(* Logix 5000 AddOnInstructionDefinition export AMCI_3202_AOP_Immediate_Stop; software revision 20.03 *)

ADD_ON_INSTRUCTION AMCI_3202_AOP_Immediate_Stop   (* revision 1.0, vendor AMCI, ExecuteEnableInFalse *)
VAR_INPUT
   channel_number : INT; {required}
END_VAR
VAR_IN_OUT
   AMCI_3202_output_data : AM:1756_3202:O:0; {required}
END_VAR
VAR
   command_data_block : DINT[8]; {access None}
END_VAR

ROUTINE EnableInFalse   (* ladder *)
END_ROUTINE

ROUTINE Logic   (* ladder *)
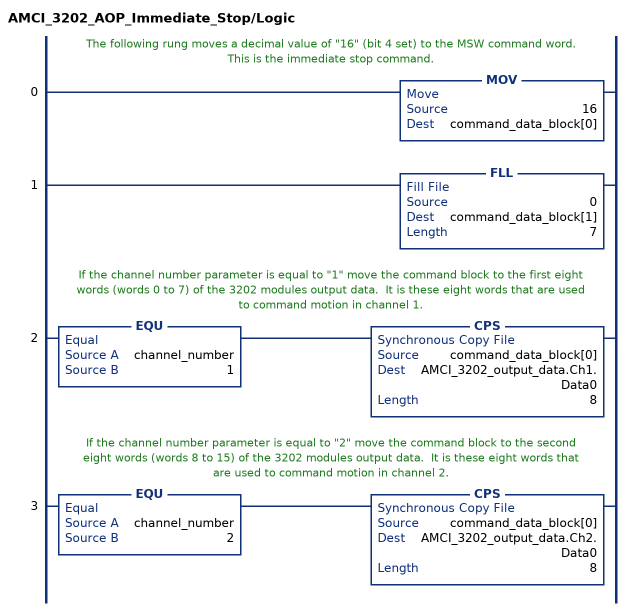
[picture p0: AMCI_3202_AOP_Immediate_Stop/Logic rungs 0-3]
   // The following rung moves a decimal value of "16" (bit 4 set) to the MSW command word.  This is the immediate stop command.
   0: MOV(16,command_data_block[0]);
   1: FLL(0,command_data_block[1],7);
   // If the channel number parameter is equal to "1" move the command block to the first eight words (words 0 to 7) of the 3202 modules output data.  It is these eight words that are used to command motion in channel 1.
   2: EQU(channel_number,1)CPS(command_data_block[0],AMCI_3202_output_data.Ch1.Data0,8);
   // If the channel number parameter is equal to "2" move the command block to the second eight words (words 8 to 15) of the 3202 modules output data.  It is these eight words that are used to command motion in channel 2.
   3: EQU(channel_number,2)CPS(command_data_block[0],AMCI_3202_output_data.Ch2.Data0,8);
END_ROUTINE
END_ADD_ON_INSTRUCTION
